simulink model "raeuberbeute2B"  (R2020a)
settings: Solver=ode45  StartTime=0.0  StopTime=1000  FixedStep=0.1  MaxStep=0.25  RelTol=1e-10  AbsTol=1e-10  EnableMultiTasking=on
InitFcn:
  | daten = load('faengeProRaeuber.csv');
libraries: simulink x1

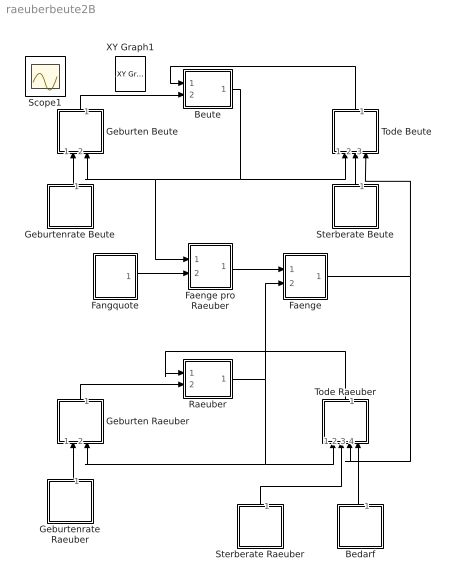
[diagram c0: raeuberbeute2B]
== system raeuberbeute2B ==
  Bedarf : Subsystem  mask{k=2}
      mask prompts: k "Constant"
  Beute : Subsystem  mask{m0=500}
      mask prompts: m0 "Anfangswert"
  Faenge : Subsystem
  Faenge pro Raeuber : Subsystem
  Fangquote : Subsystem  mask{k=0.01}
      mask prompts: k "Constant"
  Geburten Beute : Subsystem
  Geburten Raeuber : Subsystem
  Geburtenrate Beute : Subsystem  mask{k=0.2}
      mask prompts: k "Constant"
  Geburtenrate Raeuber : Subsystem  mask{k=0.1}
      mask prompts: k "Constant"
  Raeuber : Subsystem  mask{m0=20}
      mask prompts: m0 "Anfangswert"
  Sterberate Beute : Subsystem  mask{k=0.1}
      mask prompts: k "Constant"
  Sterberate Raeuber : Subsystem  mask{k=0.2}
      mask prompts: k "Constant"
  Tode Beute : Subsystem
  Tode Raeuber : Subsystem
  Scope1 : Scope
  XY Graph1 : simulink/Sinks/XY Graph  IOType=viewer  xmin=0  xmax=2300  ymin=0  ymax=1300  st=-1
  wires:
  Beute/1(Out1) -> Tode Beute/1(In1), Geburten Beute/2(In2), Faenge pro Raeuber/1(In1)
  Faenge/1(Out1) -> Tode Beute/3(In3), Tode Raeuber/3(In3)
  Raeuber/1(Out1) -> Geburten Raeuber/2(In2), Tode Raeuber/1(In1), Faenge/2(In2)
  Fangquote/1(Out1) -> Faenge pro Raeuber/2(In2)
  Geburten Beute/1(Out1) -> Beute/2(In2)
  Geburtenrate Beute/1(Out1) -> Geburten Beute/1(In1)
  Tode Beute/1(Out1) -> Beute/1(In1)
  Sterberate Beute/1(Out1) -> Tode Beute/2(In2)
  Geburten Raeuber/1(Out1) -> Raeuber/2(In2)
  Geburtenrate Raeuber/1(Out1) -> Geburten Raeuber/1(In1)
  Tode Raeuber/1(Out1) -> Raeuber/1(In1)
  Bedarf/1(Out1) -> Tode Raeuber/4(In4)
  Sterberate Raeuber/1(Out1) -> Tode Raeuber/2(In2)
  Faenge pro Raeuber/1(Out1) -> Faenge/1(In1)

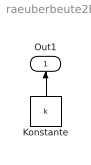
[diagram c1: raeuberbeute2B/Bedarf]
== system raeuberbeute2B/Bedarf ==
  Konstante : Constant  Value=k
  Out1 : Outport
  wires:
  Konstante/1 -> Out1/1

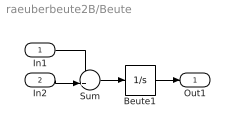
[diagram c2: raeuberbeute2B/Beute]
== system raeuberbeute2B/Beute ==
  In1 : Inport
  In2 : Inport  Port=2
  Beute1 : Integrator  InitialCondition=m0
  Sum : Sum  Inputs=-+|  SaturateOnIntegerOverflow=on
  Out1 : Outport
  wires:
  In2/1 -> Sum/2
  Beute1/1 -> Out1/1
  In1/1 -> Sum/1
  Sum/1 -> Beute1/1

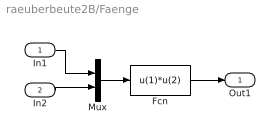
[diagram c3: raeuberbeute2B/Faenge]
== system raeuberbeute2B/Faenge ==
  In1 : Inport
  In2 : Inport  Port=2
  Fcn : Fcn  Expr=u(1)*u(2)
  Mux : Mux  Inputs=2
  Out1 : Outport
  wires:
  In2/1 -> Mux/2
  In1/1 -> Mux/1
  Mux/1 -> Fcn/1
  Fcn/1 -> Out1/1

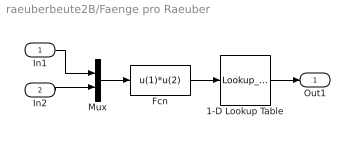
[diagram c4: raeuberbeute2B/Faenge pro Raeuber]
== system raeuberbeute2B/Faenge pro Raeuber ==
  In1 : Inport
  In2 : Inport  Port=2
  1-D Lookup Table : Lookup_n-D  NumberOfTableDimensions=1  BreakpointsForDimension1=daten(:,1)  Table=daten(:,2)  ExtrapMethod=Clip  UseLastTableValue=on  RndMeth=Simplest
  Fcn : Fcn  Expr=u(1)*u(2)
  Mux : Mux  Inputs=2
  Out1 : Outport
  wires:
  In2/1 -> Mux/2
  In1/1 -> Mux/1
  Mux/1 -> Fcn/1
  Fcn/1 -> 1-D Lookup Table/1
  1-D Lookup Table/1 -> Out1/1

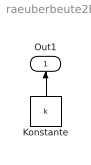
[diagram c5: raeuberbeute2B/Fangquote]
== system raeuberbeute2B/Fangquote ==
  Konstante : Constant  Value=k
  Out1 : Outport
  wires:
  Konstante/1 -> Out1/1

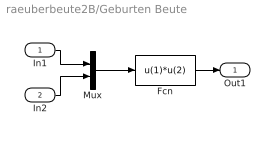
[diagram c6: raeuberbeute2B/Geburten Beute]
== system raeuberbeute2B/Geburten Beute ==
  In1 : Inport
  In2 : Inport  Port=2
  Fcn : Fcn  Expr=u(1)*u(2)
  Mux : Mux  Inputs=2
  Out1 : Outport
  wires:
  In2/1 -> Mux/2
  In1/1 -> Mux/1
  Mux/1 -> Fcn/1
  Fcn/1 -> Out1/1

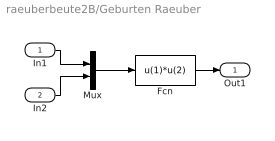
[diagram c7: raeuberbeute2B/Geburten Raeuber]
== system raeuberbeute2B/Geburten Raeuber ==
  In1 : Inport
  In2 : Inport  Port=2
  Fcn : Fcn  Expr=u(1)*u(2)
  Mux : Mux  Inputs=2
  Out1 : Outport
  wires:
  In2/1 -> Mux/2
  In1/1 -> Mux/1
  Mux/1 -> Fcn/1
  Fcn/1 -> Out1/1

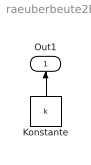
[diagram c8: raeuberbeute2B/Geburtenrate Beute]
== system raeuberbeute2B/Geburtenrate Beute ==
  Konstante : Constant  Value=k
  Out1 : Outport
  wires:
  Konstante/1 -> Out1/1

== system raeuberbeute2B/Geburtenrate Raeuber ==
  Konstante : Constant  Value=k
  Out1 : Outport
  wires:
  Konstante/1 -> Out1/1

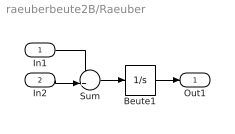
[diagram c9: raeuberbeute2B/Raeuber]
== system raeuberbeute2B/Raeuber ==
  In1 : Inport
  In2 : Inport  Port=2
  Beute1 : Integrator  InitialCondition=m0
  Sum : Sum  Inputs=-+|  SaturateOnIntegerOverflow=on
  Out1 : Outport
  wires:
  In2/1 -> Sum/2
  Beute1/1 -> Out1/1
  In1/1 -> Sum/1
  Sum/1 -> Beute1/1

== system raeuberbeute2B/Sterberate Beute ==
  Konstante : Constant  Value=k
  Out1 : Outport
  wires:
  Konstante/1 -> Out1/1

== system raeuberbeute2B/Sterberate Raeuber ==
  Konstante : Constant  Value=k
  Out1 : Outport
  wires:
  Konstante/1 -> Out1/1

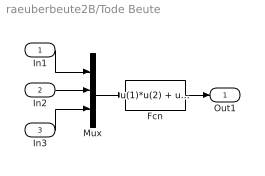
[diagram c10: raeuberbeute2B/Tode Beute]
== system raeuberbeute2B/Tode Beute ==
  In1 : Inport
  In2 : Inport  Port=2
  In3 : Inport  Port=3
  Fcn : Fcn  Expr=u(1)*u(2) + u(3)
  Mux : Mux  Inputs=3
  Out1 : Outport
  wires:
  In2/1 -> Mux/2
  In1/1 -> Mux/1
  Mux/1 -> Fcn/1
  Fcn/1 -> Out1/1
  In3/1 -> Mux/3

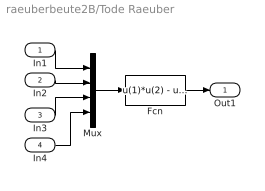
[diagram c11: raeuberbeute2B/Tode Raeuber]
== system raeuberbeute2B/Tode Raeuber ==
  In1 : Inport
  In2 : Inport  Port=2
  In3 : Inport  Port=3
  In4 : Inport  Port=4
  Fcn : Fcn  Expr=u(1)*u(2) - u(3)/u(4)
  Mux : Mux
  Out1 : Outport
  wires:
  In2/1 -> Mux/2
  In1/1 -> Mux/1
  Mux/1 -> Fcn/1
  Fcn/1 -> Out1/1
  In3/1 -> Mux/3
  In4/1 -> Mux/4
